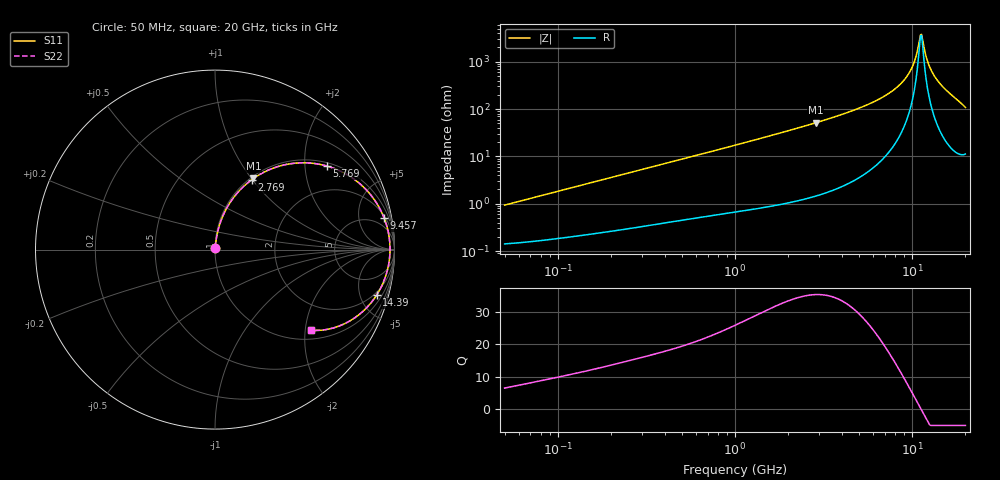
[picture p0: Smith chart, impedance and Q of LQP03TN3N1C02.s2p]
!Murata Part Number: LQP03TN3N1C02
!These Parameters are Measured in Series Mode Connection
!  o--[Z]--o
!Port1  Port2
!  o-------o
!Freq. Start=50[MHz] Stop=20[GHz], 401[Steps]
# Hz S RI R 50
!Freq.(Hz) S11(Real) S11(Imag) S21(Real) S21(Imag) S12(Real) S12(Imag) S22(Real) S22(Imag)
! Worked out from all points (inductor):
!   401 points, 50 MHz to 20 GHz, reference 50 ohm
!   read as one part in series: L = 2.93 nH near 51.52 MHz
!   highest Q = 35.4 at 2.853 GHz (marker M1), where L = 2.86 nH
!   self-resonance near 11.15 GHz
!   S11 on the Smith chart (normalised r, x): 50 MHz: 1.00, +0.02; 2.769 GHz: 1.03, +0.99; 5.769 GHz: 1.10, +2.60; 9.457 GHz: 2, +10; 14.39 GHz: 1.68, -6.83; 20 GHz: 1.22, -2.15
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5e7  0.0015 0.00921  0.9985 -0.00921  0.9985 -0.00921  0.0015 0.00921
1.364002e8  0.00274 0.0245  0.9973 -0.0245  0.9973 -0.0245  0.00274 0.0245
3.721004e8  0.00791 0.0643  0.9921 -0.0643  0.9921 -0.0643  0.00791 0.0643
1e9  0.0347 0.1648  0.9653 -0.1648  0.9653 -0.1648  0.0347 0.1648
1.766834e9  0.0927 0.275  0.9073 -0.275  0.9073 -0.275  0.0927 0.275
2.728004e9  0.1985 0.3849  0.8015 -0.3849  0.8015 -0.3849  0.1985 0.3849
2.769174e9  0.2037 0.3888  0.7963 -0.3888  0.7963 -0.3888  0.2037 0.3888
2.853386e9  0.2144 0.3965  0.7856 -0.3965  0.7856 -0.3965  0.2144 0.3965
4.275624e9  0.4134 0.4773  0.5866 -0.4773  0.5866 -0.4773  0.4134 0.4773
5.769027e9  0.6237 0.4655  0.3763 -0.4655  0.3763 -0.4655  0.6237 0.4655
7.442007e9  0.8124 0.3625  0.1876 -0.3625  0.1876 -0.3625  0.8124 0.3625
8.516016e9  0.8955 0.2668  0.1045 -0.2668  0.1045 -0.2668  0.8955 0.2668
9.457416e9  0.943 0.1748  0.057 -0.1748  0.057 -0.1748  0.943 0.1748
1.019291e10  0.9647 0.1016  0.0353 -0.1016  0.0353 -0.1016  0.9647 0.1016
1.098561e10  0.9747 0.0244  0.0253 -0.0244  0.0253 -0.0244  0.9747 0.0244
1.131968e10  0.9751 -0.00726  0.0249 0.00726  0.0249 0.00726  0.9751 -0.00726
1.149051e10  0.9746 -0.0231  0.0254 0.0231  0.0254 0.0231  0.9746 -0.0231
1.257102e10  0.9598 -0.1183  0.0402 0.1183  0.0402 0.1183  0.9598 -0.1183
1.334722e10  0.939 -0.1802  0.061 0.1802  0.061 0.1802  0.939 -0.1802
1.438523e10  0.9004 -0.2538  0.0996 0.2538  0.0996 0.2538  0.9004 -0.2538
1.670968e10  0.7803 -0.3788  0.2197 0.3788  0.2197 0.3788  0.7803 -0.3788
2e10  0.5352 -0.4494  0.4648 0.4494  0.4648 0.4494  0.5352 -0.4494
